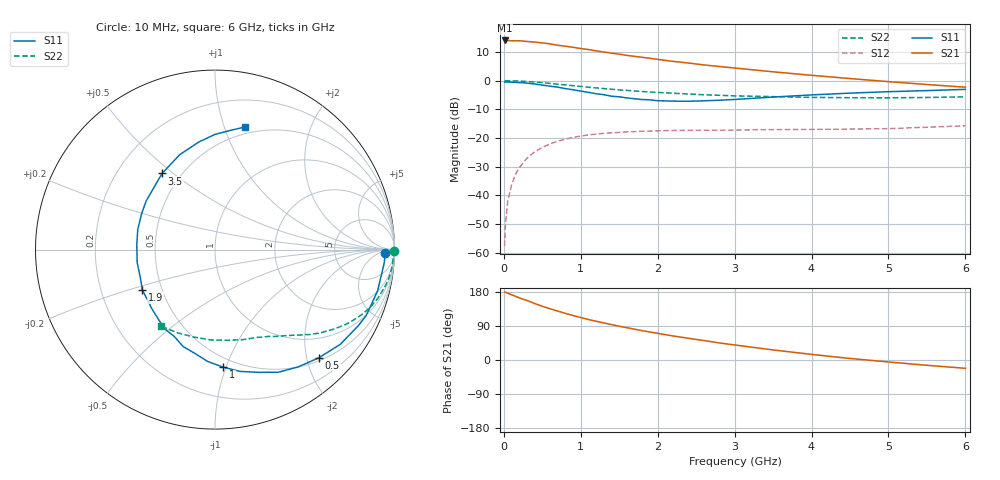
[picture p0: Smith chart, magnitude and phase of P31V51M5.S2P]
! SIEMENS Small Signal Semiconductors
! BFP181
! Si NPN RF Bipolar Junction Transistor in SOT143
! VCE = 1.5 V  IC = 1.5 mA
! Common Emitter S-Parameters:  March  1996
# GHz  S  MA  R  50
!  f  S11  S21  S12  S22
! GHz  MAG  ANG  MAG  ANG  MAG  ANG  MAG  ANG
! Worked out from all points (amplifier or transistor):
!   36 points, 10 MHz to 6 GHz, reference 50 ohm
!   highest |S21| = 14.0 dB at 10 MHz (marker M1)
!   |S21| within 3 dB of that: start of sweep to 1.051 GHz
!   unconditionally stable (mu >= 1): 2.6 GHz to end of sweep
!   at 250 MHz: K = 0.11, MSG = 21.3 dB, |S12| = -28.7 dB
!   at 1.4 GHz: K = 0.60, MSG = 13.9 dB, |S12| = -18.2 dB
!   at 6 GHz: K = 1.22, MAG = 3.9 dB, |S12| = -15.8 dB
!   S11 on the Smith chart (normalised r, x): 10 MHz: 32, -11; 500 MHz: 0.56, -2.23; 1 GHz: 0.42, -0.98; 1.9 GHz: 0.39, -0.22; 3.5 GHz: 0.39, +0.46; 6 GHz: 0.44, +1.18
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0.01  0.9453 -1.1  5.017 179.5  0.0013 99.5  0.9975 -0.4
0.02  0.9481 -1.9  4.985 179.1  0.003 86.2  0.992 -0.8
0.05  0.9456 -4.5  5.011 176.1  0.0078 91.1  0.9947 -2.2
0.1  0.9367 -9.6  4.968 172.3  0.0151 83.7  0.9925 -4.4
0.15  0.9346 -14.2  4.937 168.3  0.023 80.6  0.9889 -6.5
0.2  0.9238 -19.0  4.961 164.2  0.0302 78.5  0.9838 -8.7
0.3  0.904 -28.0  4.817 157.2  0.0444 72.5  0.9666 -12.8
0.4  0.8751 -37.1  4.7 149.1  0.0574 66.9  0.9466 -16.7
0.5  0.8359 -46.1  4.538 141.8  0.0685 61.5  0.9232 -20.4
0.6  0.8011 -54.7  4.383 135.3  0.0789 57.0  0.8951 -23.8
0.8  0.7264 -70.3  3.987 123.1  0.0955 48.3  0.8426 -29.5
1  0.6566 -86.0  3.623 112.1  0.108 41.2  0.7906 -34.3
1.1  0.6244 -93.8  3.485 106.8  0.113 38.1  0.7668 -36.4
1.3  0.5687 -108.2  3.156 97.8  0.1202 32.5  0.7264 -40.2
1.5  0.5222 -122.8  2.896 89.1  0.1252 28.2  0.6888 -43.4
1.9  0.4625 -151.1  2.452 73.8  0.1318 21.3  0.633 -49.1
2.2  0.4394 -170.8  2.165 63.4  0.1352 17.6  0.6031 -53.1
2.8  0.455 154.0  1.765 45.1  0.1369 12.4  0.5553 -61.4
3.5  0.5168 124.8  1.425 26.6  0.1401 8.7  0.5259 -72.5
4.5  0.6057 98.7  1.087 4.1  0.143 5.7  0.5041 -92.4
5.5  0.6703 82.5  0.856 -14.0  0.1543 6.0  0.5086 -114.2
6  0.7045 76.1  0.768 -21.9  0.1629 5.0  0.5218 -125.3
